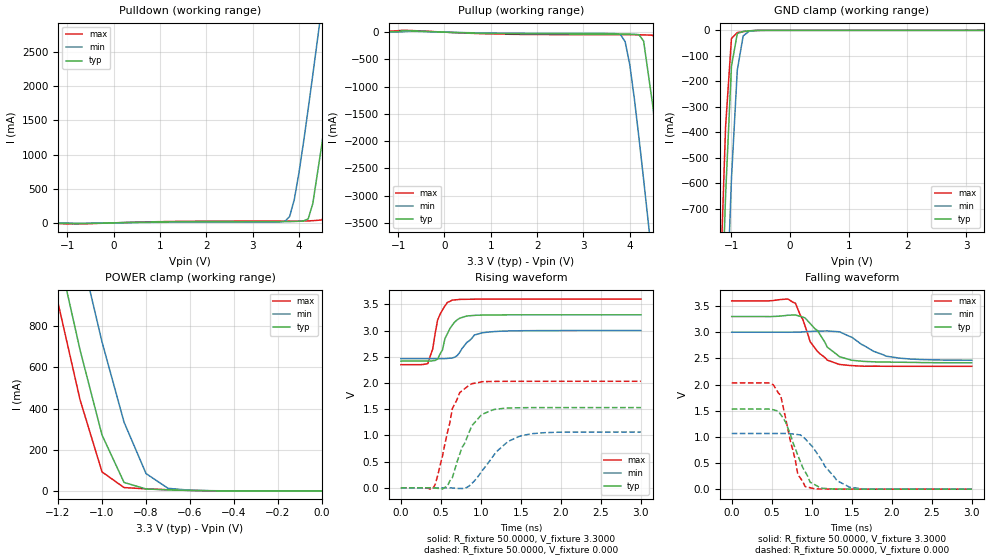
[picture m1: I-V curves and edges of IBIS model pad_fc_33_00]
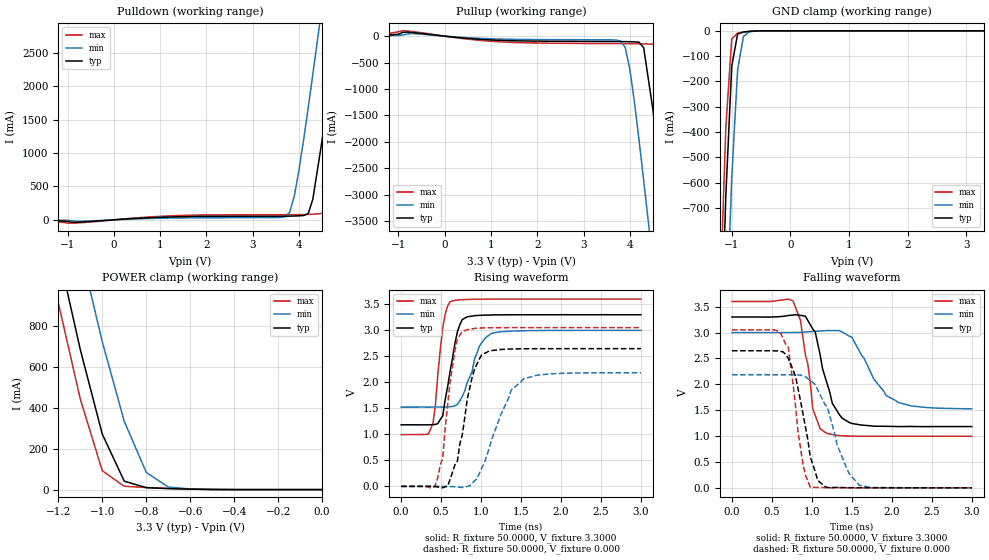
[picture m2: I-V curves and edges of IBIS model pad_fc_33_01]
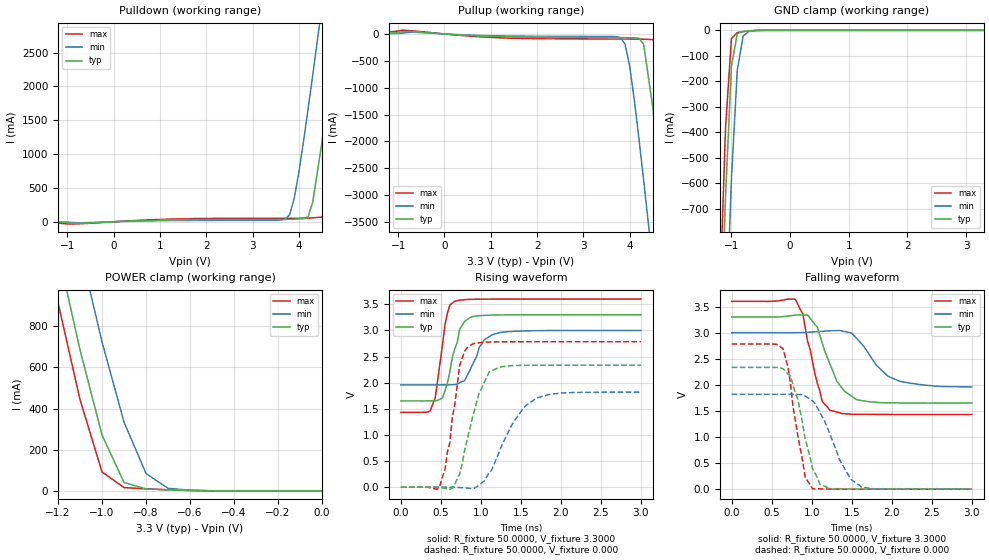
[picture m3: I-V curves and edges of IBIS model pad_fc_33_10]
| Copyright (c) 2006, Freescale.
| DISCLAIMER:
| IF FREESCALE AND THE CUSTOMER RECEIVING THIS DISCLAIMER HAVE ENTERED
| INTO AN AGREEMENT PROVIDING FOR THE NON-DISCLOSURE OR CONFIDENTIALITY OF
| INFORMATION, AND SUCH AGREEMENT COVERS THE TRANSACTION OR POTENTIAL
| TRANSACTION PURSUANT TO WHICH THE PARTIES ARE ENTERING INTO THIS
| ELECTRONIC EXCHANGE, THEN THE INFORMATION DISCLOSED HEREWITH SHALL BE
| HELD CONFIDENTIAL IN ACCORDANCE WITH THE TERMS OF SUCH AGREEMENT.
| Freescale reserves the right to make changes without further notice to
| any products herein. Freescale makes no warranty, representation or
| guarantee regarding the suitability of its products for any particular
| purpose, nor does Freescale assume any liability arising out of the
| application or use of any product or circuit, and specifically disclaims
| any and all liability, including without limitation consequential or
| incidental damages.
[IBIS Ver]   3.2
[File Name]   mcf52277mapbga196.ibs
[File Rev]   1.0
[Date]   March 13, 2008
[Source]   Data created from spice simulations by the Micro Controller
   Division, MSG, Freescale - Austin, TX
[Disclaimer]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
| Component mcf52277mapbga196
[Component]   mcf52277mapbga196.ibs
[Manufacturer]  Freescale Semiconductor Inc.
[Package]
|Units are in Ohms, Henrys and Farads.
|   typ   min   max
R_pkg   2.69E-01  1.77E-01  3.41E-01
L_pkg   6.23E-09  3.76E-09  9.22E-09
C_pkg   7.44E-13  5.29E-13  1.54E-12
[Pin] signal_name   model_name  R_pin  L_pin  C_pin
A01	LCD_D6	pad_fc
A02	LCD_D5	pad_fc
A03	LCD_D4	pad_fc
A04	LCD_D2	pad_fc
A05	LCD_LSCLK	pad_fc
A06	T0IN	pad_fc
A07	U1TXD	pad_fc
A08	U1RXD	pad_fc
A09	USB_DM	pad_ae
A10	USB_DP	pad_ae
A11	FB_CS2_b	pad_rfc
A12	FB_A21	pad_rfc
A13	FB_A17	pad_rfc
A14	FB_A16	pad_rfc
B01	LCD_D8	pad_fc
B02	LCD_D7	pad_fc
B03	LCD_D3	pad_fc
B04	LCD_D1	pad_fc
B05	LCD_ACD	pad_fc
B06	T1IN	pad_fc
B07	IRQ_1_b	pad_fc
B08	UIRTS_b	pad_fc
B09	DSPI_PCS0	pad_fc
B10	VDD_USB	POWER
B11	FB_CS3_b	pad_rfc
B12	FB_A20	pad_rfc
B13	FB_A18	pad_rfc
B14	FB_A15	pad_rfc
C01	LCD_D13	pad_fc
C02	LCD_D12	pad_fc
C03	LCD_D10	pad_fc
C04	LCD_D0	pad_fc
C05	I2C_SCO	pad_fc
C06	T2IN	pad_fc
C07	IRQ_4_b	pad_fc
C08	U1CTS_b	pad_fc
C09	DSPI_SCK	pad_fc
C10	FB_CS0_b	pad_rfc
C11	FB_A23	pad_rfc
C12	FB_A19	pad_rfc
C13	FB_A14	pad_rfc
C14	FB_A13	pad_rfc
D01	LCD_D15	pad_fc
D02	LCD_D14	pad_fc
D03	LCD_D11	pad_fc
D04	LCD_D9	pad_fc
D05	I2C_SDA	pad_fc
D06	T3IN	pad_fc
D07	IRQ_7_b	pad_fc
D08	DSPI_SIN	pad_fc
D09	DSPI_SOUT	pad_fc
D10	FB_CS1_b	pad_rfc
D11	FB_A22	pad_rfc
D12	FB_A12	pad_rfc
D13	FB_A11	pad_rfc
D14	FB_A10	pad_rfc
E01	LCD_LP	pad_fc
E02	LCD_FLM	pad_fc
E03	LCD_D17	pad_fc
E04	LCD_D16	pad_fc
E05	IVDD	POWER
E06	EVDD	POWER
E07	EVDD	POWER
E08	SDVDD	POWER
E09	SDVDD	POWER
E10	TEST	pad_fc
E11	FB_A9	pad_rfc
E12	FB_A8	pad_rfc
E13	FB_A7	pad_rfc
E14	FB_A6	pad_rfc
F01	SD_CS0_b	pad_rfc
F02	SD_CKE	pad_rfc
F03	SD_WE_b	pad_rfc
F04	FB_TS_b	pad_rfc
F05	EVDD	POWER
F06	EVDD	POWER
F07	VSS	GND
F08	VSS	GND
F09	SDVDD	POWER
F10	IVDD	POWER
F11	FB_A5	pad_rfc
F12	FB_A4	pad_rfc
F13	FB_A3	pad_rfc
F14	EXTAL	pad_ae
G01	FB_D15	pad_rfc
G02	FB_D14	pad_rfc
G03	FB_D13	pad_rfc
G04	FB_D12	pad_rfc
G05	EVDD	POWER
G06	VSS	GND
G07	VSS	GND
G08	VSS	GND
G09	SDVDD	POWER
G10	BOOTMOD1	pad_fc
G11	FB_A2	pad_rfc
G12	FB_A1	pad_rfc
G13	VDD_OSC	POWER
G14	XTAL	pad_ae
H01	FB_D11	pad_rfc
H02	FB_D10	pad_rfc
H03	FB_D9	pad_rfc
H04	FB_D8	pad_rfc
H05	SDVDD	POWER
H06	VSS	GND
H07	VSS	GND
H08	VSS	GND
H09	EVDD	POWER
H10	BOOTMOD0	pad_fc
H11	FB_A0	pad_rfc
H12	FB_TA_b	pad_rfc
H13	VSS_OSC	GND
H14	VDD_PLL	POWER
J01	FB_BWE1_b	pad_rfc
J02	SD_DQS3	pad_rfc
J03	FB_BWE3_b	pad_rfc
J04	FB_D31	pad_rfc
J05	SDVDD	POWER
J06	SDVDD	POWER
J07	VSS	GND
J08	VSS	GND
J09	EVDD	POWER
J10	IVDD	POWER
J11	RESET_b	pad_fc
J12	U0RTS_b	pad_fc
J13	VDD_RTC	POWER
J14	RTC_EXTAL	pad_fc
K01	FB_D30	pad_rfc
K02	FB_D29	pad_rfc
K03	FB_D28	pad_rfc
K04	FB_D27	pad_rfc
K05	IVDD	POWER
K06	SDVDD	POWER
K07	SDVDD	POWER
K08	EVDD	POWER
K09	EVDD	POWER
K10	JTAG_EN	pad_fc
K11	RSTOUT_b	pad_fc
K12	U0CTS_b	pad_fc
K13	U0RXD	pad_fc
K14	RTC_XTAL	pad_fc
L01	FB_D26	pad_rfc
L02	FB_D25	pad_rfc
L03	FB_D24	pad_rfc
L04	SD_A10	pad_rfc
L05	FB_D17	pad_rfc
L06	FB_BWE0_b	pad_rfc
L07	FB_D4	pad_rfc
L08	FB_D0	pad_rfc
L09	PST3	pad_fc
L10	DDATA3	pad_fc
L11	TDO	pad_fc
L12	U0TXD	pad_fc
L13	VDD_ADC	POWER
L14	VSS_ADC	GND
M01	SD_CLK	pad_rfc
M02	SD_SDR_DQS	pad_rfc
M03	FB_D23	pad_rfc
M04	FB_D20	pad_rfc
M05	FB_D16	pad_rfc
M06	FB_D7	pad_rfc
M07	FB_D3	pad_rfc
M08	FB_RW	pad_rfc
M09	PST2	pad_fc
M10	DDATA2	pad_fc
M11	TDI	pad_fc
M12	ADC_REF	pad_ae
M13	ACD_IN1	pad_ae
M14	ACD_IN0	pad_ae
N01	SD_CLK_b	pad_rfc
N02	SD_CAS_b	pad_rfc
N03	FB_D22	pad_rfc
N04	FB_D19	pad_rfc
N05	FB_BWE2_b	pad_rfc
N06	FB_D6	pad_rfc
N07	FB_D2	pad_rfc
N08	FB_OE_b	pad_rfc
N09	PST1	pad_fc
N10	DDATA1	pad_fc
N11	TMS	pad_fc
N12	ADC_IN6	pad_ae
N13	ADC_IN4	pad_ae
N14	ADC_IN2	pad_ae
P01	FB_CLK	pad_rfc
P02	SD_RAS_b	pad_rfc
P03	FB_D21	pad_rfc
P04	FB_D18	pad_rfc
P05	SD_DQS0	pad_rfc
P06	FB_D5	pad_rfc
P07	FB_D1	pad_rfc
P08	TCLK	pad_fc
P09	PST0	pad_fc
P10	DDATA0	pad_fc
P11	TRST_b	pad_fc
P12	ADC_IN7	pad_ae
P13	ADC_IN5	pad_ae
P14	ADC_IN3	pad_ae
| end pin list
|[Package Model] mcf52277.pkg
|   Model Selector
[Model Selector] pad_fc
pad_fc_33_00   - VDDE=3.3V, 10pF drive strength
pad_fc_33_01   - VDDE=3.3V, 20pF drive strength
pad_fc_33_10   - VDDE=3.3V, 30pF drive strength
pad_fc_33_11   - VDDE=3.3V, 50pF drive strength
pad_fc_33_in   - VDDE=3.3V, CMOS input mode
[Model Selector] pad_rfc
| 1.8V VDDE
Pad_rfc_00_1p8  10pF load drive
Pad_rfc_01_1p8  20pF load drive - open drain
Pad_rfc_10_1p8  30pF load drive
Pad_rfc_11_1p8  50pF load drive
Pad_rfc_in_1p8  Input Buffer
| 2.5V VDDE
Pad_rfc_00_2p5  10pF load drive
Pad_rfc_01_2p5  20pF load drive - open drain
Pad_rfc_10_2p5  30pF load drive
Pad_rfc_11_2p5  50pF load drive
Pad_rfc_in_2p5  Input Buffer
| 3.3V VDDE
Pad_rfc_00_3p3  10pF load drive
Pad_rfc_01_3p3  20pF load drive - open drain
Pad_rfc_10_3p3  30pF load drive
Pad_rfc_11_3p3  50pF load drive
Pad_rfc_in_3p3  Input Buffer
[Model Selector] pad_ae
pad_ae_33   - VDDE=3.3V, input only
| Models and submodels in the file (21): pad_fc_33_00 (3-state), pad_fc_33_01 (3-state), pad_fc_33_10 (3-state), pad_fc_33_11 (3-state), pad_fc_33_in (Input), pad_ae_33 (Input), Pad_rfc_00_1p8 (3-state), Pad_rfc_00_2p5 (3-state), Pad_rfc_00_3p3 (3-state), Pad_rfc_01_1p8 (Open_drain), Pad_rfc_01_2p5 (Open_drain), Pad_rfc_01_3p3 (Open_drain), Pad_rfc_10_1p8 (3-state), Pad_rfc_10_2p5 (3-state), Pad_rfc_10_3p3 (3-state), Pad_rfc_11_1p8 (3-state), Pad_rfc_11_2p5 (3-state), Pad_rfc_11_3p3 (3-state), Pad_rfc_in_1p8 (Input), Pad_rfc_in_2p5 (Input), Pad_rfc_in_3p3 (Input)
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|   Model pad_fc_33_00
[Model]   pad_fc_33_00
Model_type   3-state
Polarity   Non-Inverting
Enable   Active-High
C_comp   5.5000pF   5.5000pF   5.5000pF
[Temperature Range]   25.0000   0.1500k   -40.0000
[Voltage Range]   3.3000V   3.0000V   3.6000V
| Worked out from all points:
|   slope of the pulldown table from 0 to 0.495 V, typ, clamps not added: 66.6 ohm
|   slope of the pullup table from 0 to 0.495 V, typ, clamps not added: 35.1 ohm
|   GND clamp passes 1 mA (typ) near -0.63 V on its own axis
|   POWER clamp passes 1 mA (typ) near -0.52 V on its own axis
|   rising waveform, R_fixture 50.0000, V_fixture 3.3000: 20-80 % time 147ps typ, 178ps min, 118ps max; typ from 2.42 V to 3.3 V
|   rising waveform, R_fixture 50.0000, V_fixture 0.000: 20-80 % time 245ps typ, 352ps min, 195ps max; typ from 0 V to 1.53 V
|   falling waveform, R_fixture 50.0000, V_fixture 3.3000: 20-80 % time 292ps typ, 377ps min, 245ps max; typ from 3.3 V to 2.42 V
|   falling waveform, R_fixture 50.0000, V_fixture 0.000: 20-80 % time 240ps typ, 308ps min, 177ps max; typ from 1.53 V to 0 V
[Pulldown]
| voltage   I(typ)   I(min)   I(max)
-3.3V     -510uA     -300uA     -610uA
3.7V      18.38mA    23.52mA    25.96mA
3.8V      18.93mA    93.87mA    26.01mA
3.9V      20.66mA    341.7mA    26.07mA
4.2V      58.16mA    1.668A     28.58mA
4.3V      283.6mA    2.169A     31.96mA
4.5V      1.172A     3.192A     42.6mA
4.7V      2.193A     4.227A     458.6mA
4.9V      3.242A     5.265A     1.434A
5.1V      4.299A     6.306A     2.483A
5.3V      5.359A     7.347A     3.548A
6.6V      12.26A     14.12A     10.52A
[Pullup]
| voltage   I(typ)   I(min)   I(max)
-3.3V     1.1mA      1.1mA      1.1mA
-900mV    24.08mA    7.447mA    34.76mA
3.8V      -34.2mA    -44.36mA   -47.19mA
3.9V      -34.79mA   -173.2mA   -47.31mA
4V        -36.28mA   -595mA     -47.43mA
4.2V      -46.68mA   -1.949A    -48.23mA
4.3V      -166.4mA   -2.709A    -50.07mA
4.5V      -1.366A    -4.279A    -56.77mA
4.7V      -2.932A    -5.872A    -403.2mA
4.9V      -4.554A    -7.469A    -1.856A
5.1V      -6.191A    -9.067A    -3.48A
6.6V      -18.48A    -21.05A    -15.94A
[GND_clamp]
| voltage   I(typ)   I(min)   I(max)
-3.3V     -18.48A    -18.65A    -18.42A
-1.2V     -1.357A    -1.942A    -1.067A
-1.1V     -650.5mA   -1.219A    -380mA
-1V       -141.2mA   -584.4mA   -32.29mA
-900mV    -12.85mA   -155.8mA   -8.89mA
-800mV    -4.42mA    -21.92mA   -5.229mA
-700mV    -2.049mA   -3.904mA   -2.397mA
-400mV    -7.776uA   -47.99uA   -2.574uA
3.3V      2.182uA    34.68uA    1.661uA
[POWER_clamp]
| voltage   I(typ)   I(min)   I(max)
-3.3V     12.25A     12.55A     12.11A
-1.3V     1.667A     2.163A     1.421A
-1.2V     1.163A     1.662A     913.9mA
-1.1V     684.8mA    1.177A     443.1mA
-1V       271.3mA    723.4mA    92.34mA
-900mV    41.22mA    334.1mA    16.32mA
-800mV    9.5mA      84.35mA    10.09mA
-700mV    5.131mA    12.62mA    5.713mA
-600mV    2.291mA    3.317mA    2.385mA
-500mV    581uA      1.097mA    477.4uA
0V        2.182uA    2.618uA    2.249uA
[Ramp]
| variable   typ   min   max
dV/dt_r   0.9182/0.2515n   0.6384/0.3474n   1.2192/0.1995n
dV/dt_f   0.5300/0.2893n   0.3211/0.3785n   0.7509/0.2422n
R_load = 50.0000
[Rising Waveform]
R_fixture = 50.0000
V_fixture = 3.3000
V_fixture_min = 3.0000
V_fixture_max = 3.6000
| time   V(typ)   V(min)   V(max)
0s        2.417V     2.463V     2.348V
336.7ps   2.417V     2.463V     2.367V
398ps     2.423V     2.463V     2.647V
459.2ps   2.455V     2.463V     3.199V
581.6ps   2.94V      2.468V     3.536V
642.9ps   3.103V     2.476V     3.58V
734.7ps   3.234V     2.581V     3.593V
918.4ps   3.288V     2.914V     3.598V
1.01ns    3.294V     2.955V     3.598V
3ns       3.3V       2.999V     3.6V
[Rising Waveform]
R_fixture = 50.0000
V_fixture = 0.000
| time   V(typ)   V(min)   V(max)
0s        2.217nV    763.3nV    91.55pV
398ps     -1.205mV   29.65uV    -17.44mV
520.4ps   -21.9mV    675uV      608.1mV
642.9ps   190.9mV    -3.18mV    1.508V
734.7ps   638.8mV    -12.05mV   1.814V
887.8ps   1.184V     84.83mV    1.986V
1.133ns   1.476V     561.3mV    2.028V
1.316ns   1.52V      853.7mV    2.031V
1.5ns     1.527V     990.8mV    2.031V
3ns       1.53V      1.064V     2.032V
[Falling Waveform]
R_fixture = 50.0000
V_fixture = 3.3000
V_fixture_min = 3.0000
V_fixture_max = 3.6000
| time   V(typ)   V(min)   V(max)
0s        3.3V       3V         3.6V
704.1ps   3.325V     2.999V     3.634V
795.9ps   3.33V      3.002V     3.555V
887.8ps   3.29V      3.006V     3.249V
979.6ps   3.168V     3.015V     2.822V
1.071ns   3.033V     3.021V     2.633V
1.194ns   2.716V     3.024V     2.468V
1.347ns   2.532V     3.008V     2.384V
1.929ns   2.429V     2.542V     2.349V
3ns       2.417V     2.465V     2.348V
[Falling Waveform]
R_fixture = 50.0000
V_fixture = 0.000
| time   V(typ)   V(min)   V(max)
0s        1.53V      1.064V     2.032V
520.4ps   1.518V     1.064V     1.996V
612.2ps   1.426V     1.064V     1.791V
826.5ps   648.9mV    1.043V     281.5mV
918.4ps   332.7mV    962.5mV    49.76mV
979.6ps   133.4mV    860.2mV    27.91mV
1.102ns   32.99mV    604.4mV    3.664mV
1.316ns   2.738mV    161.7mV    802.4uV
1.469ns   1.405mV    38.16mV    230.8uV
3ns       2.543uV    41.89uV    1.132uV
|   Model pad_fc_33_01
[Model]   pad_fc_33_01
Model_type   3-state
Polarity   Non-Inverting
Enable   Active-High
C_comp   5.5000pF   5.5000pF   5.5000pF
[Temperature Range]   25.0000   0.1500k   -40.0000
[Voltage Range]   3.3000V   3.0000V   3.6000V
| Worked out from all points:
|   slope of the pulldown table from 0 to 0.495 V, typ, clamps not added: 22.2 ohm
|   slope of the pullup table from 0 to 0.495 V, typ, clamps not added: 11.7 ohm
|   GND clamp passes 1 mA (typ) near -0.63 V on its own axis
|   POWER clamp passes 1 mA (typ) near -0.52 V on its own axis
|   rising waveform, R_fixture 50.0000, V_fixture 3.3000: 20-80 % time 146ps typ, 192ps min, 99.4ps max; typ from 1.18 V to 3.3 V
|   rising waveform, R_fixture 50.0000, V_fixture 0.000: 20-80 % time 185ps typ, 320ps min, 132ps max; typ from 0 V to 2.65 V
|   falling waveform, R_fixture 50.0000, V_fixture 3.3000: 20-80 % time 206ps typ, 344ps min, 142ps max; typ from 3.3 V to 1.18 V
|   falling waveform, R_fixture 50.0000, V_fixture 0.000: 20-80 % time 194ps typ, 300ps min, 145ps max; typ from 2.65 V to 0 V
[Pulldown]
| voltage   I(typ)   I(min)   I(max)
-3.3V     -1.53mA    -910uA     -1.86mA
3.7V      55.03mA    45.39mA    77.86mA
3.8V      55.64mA    113.1mA    78.03mA
3.9V      57.42mA    356.8mA    78.21mA
4.2V      92.35mA    1.679A     81.01mA
4.3V      308.3mA    2.18A      84.49mA
4.5V      1.192A     3.203A     95.24mA
4.7V      2.212A     4.238A     489.4mA
4.9V      3.26A      5.277A     1.46A
5.1V      4.317A     6.317A     2.509A
5.3V      5.377A     7.359A     3.574A
6.6V      12.28A     14.13A     10.55A
[Pullup]
| voltage   I(typ)   I(min)   I(max)
-3.3V     3.8mA      3.8mA      3.8mA
-900mV    73.55mA    23.56mA    105mA
1.2V      -79.48mA   -55mA      -107.4mA
3.8V      -102.4mA   -89.56mA   -141.6mA
3.9V      -103.2mA   -209.8mA   -142mA
4V        -104.8mA   -619.6mA   -142.3mA
4.3V      -219.1mA   -2.725A    -145.5mA
4.5V      -1.391A    -4.293A    -152.6mA
4.7V      -2.952A    -5.886A    -454.5mA
4.9V      -4.574A    -7.483A    -1.885A
5.1V      -6.21A     -9.081A    -3.507A
6.6V      -18.5A     -21.06A    -15.96A
[GND_clamp]
| voltage   I(typ)   I(min)   I(max)
-3.3V     -18.48A    -18.65A    -18.42A
-1.2V     -1.357A    -1.942A    -1.067A
-1.1V     -650.5mA   -1.219A    -380mA
-1V       -141.2mA   -584.4mA   -32.29mA
-900mV    -12.85mA   -155.8mA   -8.89mA
-800mV    -4.42mA    -21.92mA   -5.229mA
-700mV    -2.049mA   -3.904mA   -2.397mA
-400mV    -7.776uA   -47.99uA   -2.574uA
3.3V      2.182uA    34.68uA    1.661uA
[POWER_clamp]
| voltage   I(typ)   I(min)   I(max)
-3.3V     12.25A     12.55A     12.11A
-1.3V     1.667A     2.163A     1.421A
-1.2V     1.163A     1.662A     913.9mA
-1.1V     684.8mA    1.177A     443.1mA
-1V       271.3mA    723.4mA    92.34mA
-900mV    41.22mA    334.1mA    16.32mA
-800mV    9.5mA      84.35mA    10.09mA
-700mV    5.131mA    12.62mA    5.713mA
-600mV    2.291mA    3.317mA    2.385mA
-500mV    581uA      1.097mA    477.4uA
0V        2.182uA    2.618uA    2.249uA
[Ramp]
| variable   typ   min   max
dV/dt_r   1.5887/0.1977n   1.3106/0.3265n   1.8314/0.1390n
dV/dt_f   1.2701/0.2233n   0.8836/0.3528n   1.5627/0.1557n
R_load = 50.0000
[Rising Waveform]
R_fixture = 50.0000
V_fixture = 3.3000
V_fixture_min = 3.0000
V_fixture_max = 3.6000
| time   V(typ)   V(min)   V(max)
0s        1.183V     1.524V     995.5mV
336.7ps   1.184V     1.524V     1.001V
398ps     1.187V     1.524V     1.211V
520.4ps   1.355V     1.525V     3.047V
612.2ps   2.207V     1.532V     3.549V
704.1ps   2.973V     1.578V     3.581V
765.3ps   3.208V     1.73V      3.589V
979.6ps   3.287V     2.697V     3.598V
1.133ns   3.295V     2.943V     3.599V
3ns       3.3V       3V         3.6V
[Rising Waveform]
R_fixture = 50.0000
V_fixture = 0.000
| time   V(typ)   V(min)   V(max)
0s        1.145nV    442.2nV    44.06pV
428.6ps   -5.033mV   122uV      25.1mV
520.4ps   -26.69mV   516.7uV    544.9mV
581.6ps   2.601mV    -923.4uV   1.562V
673.5ps   416.9mV    -7.611mV   2.619V
765.3ps   993.8mV    -21.68mV   2.982V
887.8ps   2.093V     57.43mV    3.028V
1.01ns    2.537V     358.4mV    3.046V
1.531ns   2.645V     2.066V     3.052V
3ns       2.648V     2.184V     3.052V
[Falling Waveform]
R_fixture = 50.0000
V_fixture = 3.3000
V_fixture_min = 3.0000
V_fixture_max = 3.6000
| time   V(typ)   V(min)   V(max)
0s        3.3V       3V         3.6V
765.3ps   3.338V     3.001V     3.608V
857.1ps   3.331V     3.003V     3.239V
949ps     3.234V     3.013V     2.391V
1.01ns    3.069V     3.019V     1.533V
1.163ns   2.149V     3.036V     1.074V
1.255ns   1.632V     3.038V     1.03V
1.5ns     1.243V     2.909V     999.3mV
1.929ns   1.188V     1.784V     995.6mV
3ns       1.183V     1.527V     995.5mV
[Falling Waveform]
R_fixture = 50.0000
V_fixture = 0.000
| time   V(typ)   V(min)   V(max)
0s        2.648V     2.185V     3.052V
551ps     2.646V     2.185V     3.045V
704.1ps   2.504V     2.186V     2.718V
795.9ps   2.149V     2.181V     1.565V
887.8ps   1.433V     2.166V     460.2mV
979.6ps   596.1mV    2.074V     14.97mV
1.163ns   24.68mV    1.61V      4.168mV
1.439ns   2.427mV    364.8mV    753.2uV
1.592ns   1.339mV    50.19mV    -175uV
3ns       1.066uV    118.6uV    -171.9nV
|   Model Pad_fc_10
[Model]   pad_fc_33_10
Model_type   3-state
Polarity   Non-Inverting
Enable   Active-High
C_comp   5.5000pF   5.5000pF   5.5000pF
[Temperature Range]   25.0000   0.1500k   -40.0000
[Voltage Range]   3.3000V   3.0000V   3.6000V
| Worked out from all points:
|   slope of the pulldown table from 0 to 0.495 V, typ, clamps not added: 33.3 ohm
|   slope of the pullup table from 0 to 0.495 V, typ, clamps not added: 17.5 ohm
|   GND clamp passes 1 mA (typ) near -0.63 V on its own axis
|   POWER clamp passes 1 mA (typ) near -0.52 V on its own axis
|   rising waveform, R_fixture 50.0000, V_fixture 3.3000: 20-80 % time 150ps typ, 192ps min, 116ps max; typ from 1.65 V to 3.3 V
|   rising waveform, R_fixture 50.0000, V_fixture 0.000: 20-80 % time 232ps typ, 361ps min, 155ps max; typ from 0 V to 2.33 V
|   falling waveform, R_fixture 50.0000, V_fixture 3.3000: 20-80 % time 259ps typ, 333ps min, 193ps max; typ from 3.3 V to 1.65 V
|   falling waveform, R_fixture 50.0000, V_fixture 0.000: 20-80 % time 210ps typ, 316ps min, 170ps max; typ from 2.33 V to 0 V
[Pulldown]
| voltage   I(typ)   I(min)   I(max)
-3.3V     -970uA     -580uA     -1.18mA
3.7V      36.71mA    34.53mA    51.91mA
3.8V      37.29mA    104mA      52.02mA
3.9V      39.06mA    350.7mA    52.14mA
4.2V      75.74mA    1.676A     54.82mA
4.3V      298.6mA    2.177A     58.26mA
4.5V      1.186A     3.2A       68.99mA
4.7V      2.207A     4.235A     479.2mA
4.9V      3.256A     5.274A     1.454A
5.1V      4.313A     6.314A     2.503A
5.3V      5.373A     7.355A     3.568A
6.6V      12.27A     14.13A     10.54A
[Pullup]
| voltage   I(typ)   I(min)   I(max)
-3.3V     2mA        2mA        2mA
-900mV    48.64mA    15.33mA    70mA
3.8V      -68.33mA   -67.11mA   -94.41mA
3.9V      -68.99mA   -192.8mA   -94.64mA
4V        -70.55mA   -610.2mA   -94.87mA
4.1V      -73.03mA   -1.24A     -95.15mA
4.3V      -194.1mA   -2.722A    -97.82mA
4.5V      -1.384A    -4.291A    -104.8mA
4.7V      -2.949A    -5.884A    -432.8mA
4.9V      -4.571A    -7.481A    -1.879A
5.1V      -6.208A    -9.079A    -3.503A
6.6V      -18.5A     -21.06A    -15.96A
[GND_clamp]
| voltage   I(typ)   I(min)   I(max)
-3.3V     -18.48A    -18.65A    -18.42A
-1.2V     -1.357A    -1.942A    -1.067A
-1.1V     -650.5mA   -1.219A    -380mA
-1V       -141.2mA   -584.4mA   -32.29mA
-900mV    -12.85mA   -155.8mA   -8.89mA
-800mV    -4.42mA    -21.92mA   -5.229mA
-700mV    -2.049mA   -3.904mA   -2.397mA
-400mV    -7.776uA   -47.99uA   -2.574uA
3.3V      2.182uA    34.68uA    1.661uA
[POWER_clamp]
| voltage   I(typ)   I(min)   I(max)
-3.3V     12.25A     12.55A     12.11A
-1.3V     1.667A     2.163A     1.421A
-1.2V     1.163A     1.662A     913.9mA
-1.1V     684.8mA    1.177A     443.1mA
-1V       271.3mA    723.4mA    92.34mA
-900mV    41.22mA    334.1mA    16.32mA
-800mV    9.5mA      84.35mA    10.09mA
-700mV    5.131mA    12.62mA    5.713mA
-600mV    2.291mA    3.317mA    2.385mA
-500mV    581uA      1.097mA    477.4uA
0V        2.182uA    2.618uA    2.249uA
[Ramp]
| variable   typ   min   max
dV/dt_r   1.4008/0.2236n   1.0914/0.3702n   1.6699/0.1572n
dV/dt_f   0.9894/0.2627n   0.6241/0.3284n   1.3006/0.1949n
R_load = 50.0000
[Rising Waveform]
R_fixture = 50.0000
V_fixture = 3.3000
V_fixture_min = 3.0000
V_fixture_max = 3.6000
| time   V(typ)   V(min)   V(max)
0s        1.651V     1.957V     1.432V
367.3ps   1.652V     1.957V     1.464V
428.6ps   1.654V     1.957V     1.712V
520.4ps   1.712V     1.957V     2.726V
581.6ps   1.995V     1.958V     3.33V
673.5ps   2.642V     1.964V     3.559V
795.9ps   3.172V     2.037V     3.588V
979.6ps   3.282V     2.681V     3.598V
1.163ns   3.294V     2.929V     3.599V
3ns       3.3V       2.999V     3.6V
[Rising Waveform]
R_fixture = 50.0000
V_fixture = 0.000
| time   V(typ)   V(min)   V(max)
0s        1.513nV    560.5nV    59.6pV
489.8ps   -8.384mV   538.8uV    39.08mV
612.2ps   -37.9mV    -39.76uV   856.8mV
734.7ps   248.6mV    -7.402mV   2.332V
887.8ps   1.293V     -28.11mV   2.733V
979.6ps   1.808V     44.62mV    2.765V
1.102ns   2.201V     272.4mV    2.779V
1.408ns   2.327V     1.247V     2.783V
1.684ns   2.333V     1.692V     2.783V
3ns       2.335V     1.819V     2.783V
[Falling Waveform]
R_fixture = 50.0000
V_fixture = 3.3000
V_fixture_min = 3.0000
V_fixture_max = 3.6000
| time   V(typ)   V(min)   V(max)
0s        3.3V       3V         3.6V
795.9ps   3.337V     3V         3.641V
887.8ps   3.34V      3.003V     3.367V
1.071ns   3.104V     3.02V      2.025V
1.133ns   2.797V     3.026V     1.679V
1.225ns   2.412V     3.035V     1.515V
1.316ns   2.063V     3.04V      1.477V
1.561ns   1.715V     2.891V     1.435V
2.082ns   1.654V     2.08V      1.433V
3ns       1.651V     1.96V      1.432V
[Falling Waveform]
R_fixture = 50.0000
V_fixture = 0.000
| time   V(typ)   V(min)   V(max)
0s        2.335V     1.819V     2.783V
642.9ps   2.31V      1.819V     2.69V
704.1ps   2.204V     1.82V      2.336V
826.5ps   1.73V      1.815V     1.026V
918.4ps   963.2mV    1.788V     230mV
1.01ns    394.2mV    1.691V     8.552mV
1.225ns   13.25mV    1.065V     2.356mV
1.469ns   2.73mV     242.2mV    177.1uV
1.622ns   1.023mV    35.58mV    95.32uV
3ns       1.803uV    56.97uV    283.1nV
